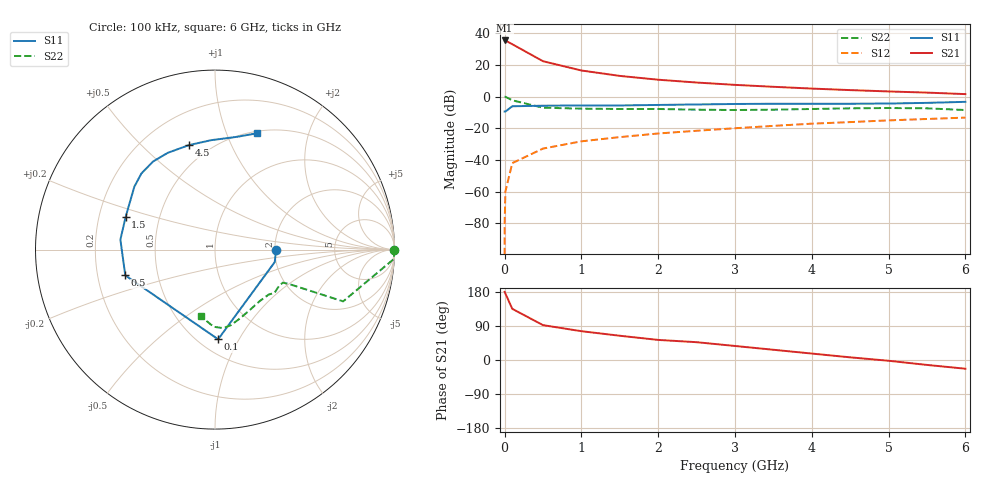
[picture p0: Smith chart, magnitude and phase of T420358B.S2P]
!AT-42035
!S-PARAMETERS at Vce=8V  Ic=35mA.  LAST UPDATED 07-21-92
# ghz s ma r 50
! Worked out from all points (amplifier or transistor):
!   16 points, 100 kHz to 6 GHz, reference 50 ohm
!   highest |S21| = 35.6 dB at 100 kHz (marker M1)
!   |S21| within 3 dB of that: start of sweep to 123.2 MHz
!   unconditionally stable (mu >= 1): start of sweep to 149.9 kHz; 878.6 MHz to 3.572 GHz
!   at 10 MHz: K = 0.02, MSG = 47.8 dB, |S12| = -60.0 dB
!   at 2.5 GHz: K = 1.11, MAG = 13.2 dB, |S12| = -21.5 dB
!   at 6 GHz: K = 0.77, MSG = 7.4 dB, |S12| = -13.2 dB
!   S11 on the Smith chart (normalised r, x): 100 kHz: 2.03, -0.00; 100 MHz: 0.62, -0.82; 500 MHz: 0.32, -0.13; 1.5 GHz: 0.32, +0.16; 4.5 GHz: 0.39, +0.71; 6 GHz: 0.52, +1.29
0.0001  0.34 -0.1  60 179.9  1e-05 86.0  0.999 0.0
0.001  0.34 -1.2  60 179.5  0.0001 89.0  0.999 -0.3
0.01  0.34 -11.8  60 175.5  0.001 87.0  0.998 -3.0
0.1  0.5 -88.0  45.64 135.0  0.008 68.0  0.77 -22.0
0.5  0.52 -164.0  13.24 92.0  0.023 57.0  0.45 -25.0
1  0.53 174.0  6.75 76.0  0.039 63.0  0.42 -26.0
1.5  0.53 160.0  4.55 64.0  0.053 66.0  0.41 -30.0
2  0.55 148.0  3.45 53.0  0.069 65.0  0.41 -36.0
2.5  0.57 142.0  2.81 47.0  0.084 67.0  0.39 -40.0
3  0.59 134.0  2.37 37.0  0.101 64.0  0.38 -49.0
3.5  0.6 125.0  2.06 27.0  0.12 61.0  0.39 -61.0
4  0.6 116.0  1.81 17.0  0.141 57.0  0.41 -71.0
4.5  0.6 104.0  1.62 7.0  0.158 50.0  0.43 -78.0
5  0.61 92.0  1.47 -2.0  0.179 45.0  0.44 -84.0
5.5  0.64 79.0  1.35 -13.0  0.198 37.0  0.43 -91.0
6  0.69 70.0  1.21 -23.0  0.219 30.0  0.38 -102.0
